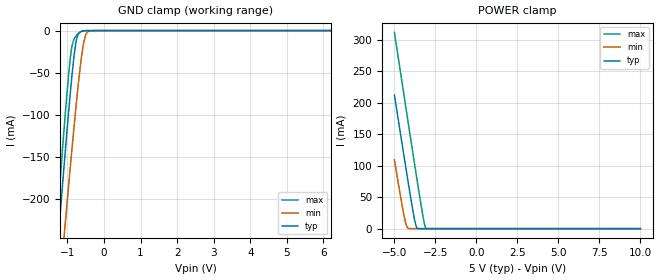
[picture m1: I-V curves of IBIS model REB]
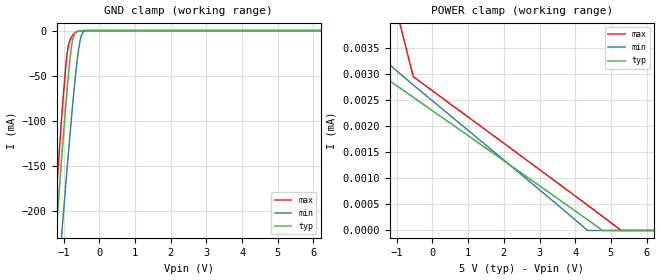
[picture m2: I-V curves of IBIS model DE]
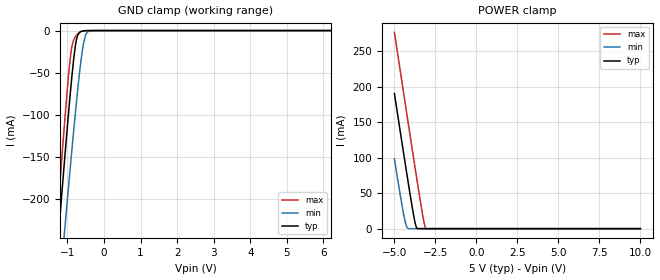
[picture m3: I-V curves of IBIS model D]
|Texas Instruments Incorporated
| THVD1550 5-V RS-485 Transceivers With +/-16-kV IEC ESD Protection
| Marketing part#   Digital Voltage Range   Package-type   #pins
| THVD1550D   4.5V-5.5V   SOIC   8
| THVD1550DGK   4.5V-5.5V   VSSOP   8
[IBIS Ver]   4.1
[File name]   thvd1550.ibs
[Date]   05/26/2017
[File Rev]   1.0
[Source]
| Texas Instruments Incorporated.
| Analog-eLab Design Center, HPA
| 12500 TI Blvd
| Dallas, TX -75243
[Notes]
| Rev 1.0: 05/26/2017
| - Initial version of the model
| - Model generated from simulations in SPECTRE
| - Model matched to SPICE simulation
| - C_comp although listed in numerical order of value are
|   obtained from varying PVT conditions. For PVT conditions for
|   each specific value refer the buffer description under
|   respective [Model]. IBIS model user is responsible for using
|   appropriate C_comp to simulate for Signal Integrity.
[Disclaimer]
| This model is designed as an aid for customers of Texas Instruments.
| TI and its licensors and suppliers make no warranties, either expressed
| or implied, with respect to this  model, including the warranties of
| merchantability or fitness for a particular purpose. The model is
| provided solely on an "as is" basis. The entire risk as to its quality
| and performance is with the customer.
[Copyright]
(C) Copyright 2017 Texas Instruments Incorporated.All rights reserved.
|   THVD1550D
[Component]   THVD1550D
[Manufacturer]  TI
[Package]   |8 SOIC - D package
|   typ   min   max
R_pkg   0   0   0
L_pkg   0   0   0
C_pkg   0   0   0
[Pin]  signal_name model_name   R_pin   L_pin   C_pin
1   R   R   NA   NA   NA
2   _RE   REB   NA   NA   NA
3   DE   DE   NA   NA   NA
4   D   D   NA   NA   NA
5   GND   gnd   NA   NA   NA
6   A   diff   NA   NA   NA
7   B   diff   NA   NA   NA
8   VCC   power   NA   NA   NA
[Diff Pin]  inv_pin  vdiff  tdelay_typ tdelay_min tdelay_max
6   7   0.2   NA   NA   NA
|   THVD1550DGK
[Component]   THVD1550DGK
[Manufacturer]  TI
[Package]   |8 VSSOP - DGK package
|   typ   min   max
R_pkg   0   0   0
L_pkg   0   0   0
C_pkg   0   0   0
[Pin]  signal_name model_name   R_pin   L_pin   C_pin
1   R   R   NA   NA   NA
2   _RE   REB   NA   NA   NA
3   DE   DE   NA   NA   NA
4   D   D   NA   NA   NA
5   GND   gnd   NA   NA   NA
6   A   diff   NA   NA   NA
7   B   diff   NA   NA   NA
8   VCC   power   NA   NA   NA
[Diff Pin]  inv_pin  vdiff  tdelay_typ tdelay_min tdelay_max
6   7   0.2   NA   NA   NA
| Models and submodels in the file (5): REB (Input), DE (Input), D (Input), R (3-state), diff (I/O)
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|   REB Model
[Model]   REB
Model_type   Input
Vinl = 0.5
Vinh = 4.5
|   typ   min   max
C_comp   6.491E-12   5.789E-12   6.939E-12
[Model spec]
|subparameter
Vinl   0.5   0.45   0.55
Vinh   4.5   4.05   4.95
| Where Nom  PVT is Nominal Process, 5V, 27C
|   Fast PVT is Strong Process,  5.5V, -40C
|   Slow PVT is Weak Process,   4.5, 150C
[Voltage Range]   5   4.5   5.5
|Junction Temperature
[Temperature Range]   27   150   -40
[Power Clamp Reference]   5   4.5   5.5
[GND Clamp Reference]   0   0   0
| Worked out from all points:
|   GND clamp passes 1 mA (typ) near -0.62 V on its own axis
|   POWER clamp passes 1 mA (typ) near -3.62 V on its own axis
[GND Clamp]
|   Voltage   I(typ)   I(min)   I(max)
-5V       -2.374A    -2.283A    -2.497A
-1.445V   -351.6mA   -421.6mA   -320.8mA
-1.25V    -244.6mA   -322.9mA   -205.9mA
-1.235V   -236.5mA   -315.3mA   -197.2mA
-1.13V    -180.1mA   -262.9mA   -137.2mA
-1.055V   -140.6mA   -225.9mA   -95.96mA
-905mV    -66.08mA   -153.6mA   -26.41mA
-770mV    -14.61mA   -91.73mA   -6.602mA
-620mV    -1.012mA   -32.37mA   -1.047mA
-485mV    -90.93uA   -3.793mA   -69.28uA
-245mV    -2.701uA   -14.54uA   -2.873uA
10V       0A         0A         0A
[POWER Clamp]
|   Voltage   I(typ)   I(min)   I(max)
-5V       212.6mA    109.6mA    312.1mA
-4.535V   135mA      37.57mA    232.5mA
-4.4V     112.7mA    19.02mA    209.4mA
-4.295V   95.5mA     7.406mA    191.5mA
-4.145V   71.14mA    530.5uA    166mA
-3.86V    26.73mA    342.2nA    117.8mA
-3.71V    7.131mA    36.81nA    92.61mA
-3.59V    443.9uA    20.17nA    72.65mA
-3.245V   0A         0A         17.76mA
-3.155V   0A         0A         6.049mA
-3.065V   0A         0A         462.9uA
10V       0A         0A         0A
|   DE Model
[Model]   DE
Model_type   Input
Vinl = 0.5
Vinh = 4.5
|   typ   min   max
C_comp   4.694E-12   4.505E-12   4.916E-12
[Model spec]
|subparameter
Vinl   0.5   0.45   0.55
Vinh   4.5   4.05   4.95
| Where Nom  PVT is Nominal Process, 5V, 27C
|   Fast PVT is Strong Process,  5.5V, -40C
|   Slow PVT is Weak Process,   4.5, 150C
[Voltage Range]   5   4.5   5.5
|Junction Temperature
[Temperature Range]   27   150   -40
[Power Clamp Reference]   5   4.5   5.5
[GND Clamp Reference]   0   0   0
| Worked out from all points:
|   GND clamp passes 1 mA (typ) near -0.62 V on its own axis
[GND Clamp]
|   Voltage   I(typ)   I(min)   I(max)
-3.6V     -1.572A    -1.544A    -1.635A
-1.319V   -281.9mA   -357.3mA   -245.9mA
-1.209V   -222.2mA   -302.1mA   -182mA
-1.05V    -138.1mA   -223.5mA   -93.32mA
-903.8mV  -65.44mA   -152.9mA   -25.92mA
-855mV    -43.85mA   -130mA     -14.31mA
-769.6mV  -14.41mA   -91.45mA   -6.57mA
-696.4mV  -3.663mA   -60.55mA   -3.123mA
-635.4mV  -1.292mA   -37.49mA   -1.345mA
-513.4mV  -153.7uA   -6.74mA    -127.1uA
-354.8mV  -5.531uA   -160.9uA   -2.275uA
8.6V      0A         0A         0A
[POWER Clamp]
|   Voltage   I(typ)   I(min)   I(max)
-3.6V     287.8uA    4.691uA    64.82mA
-3.222V   3.835uA    4.363uA    11.88mA
-2.99V    3.725uA    4.219uA    9.58uA
-537.8mV  2.553uA    2.79uA     2.948uA
2.707V    998.1nA    947.1nA    1.315uA
4.342V    207.3nA    867.5pA    486.3nA
4.757V    3.159nA    0A         274.4nA
5.306V    0A         0A         0A
8.6V      0A         0A         0A
|   D Model
[Model]   D
Model_type   Input
Vinl = 0.5
Vinh = 4.5
|   typ   min   max
C_comp   4.697E-12   4.504E-12   4.921E-12
[Model spec]
|subparameter
Vinl   0.5   0.45   0.55
Vinh   4.5   4.05   4.95
| Where Nom  PVT is Nominal Process, 5V, 27C
|   Fast PVT is Strong Process,  5.5V, -40C
|   Slow PVT is Weak Process,   4.5, 150C
[Voltage Range]   5   4.5   5.5
|Junction Temperature
[Temperature Range]   27   150   -40
[Power Clamp Reference]   5   4.5   5.5
[GND Clamp Reference]   0   0   0
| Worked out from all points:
|   GND clamp passes 1 mA (typ) near -0.62 V on its own axis
|   POWER clamp passes 1 mA (typ) near -3.64 V on its own axis
[GND Clamp]
|   Voltage   I(typ)   I(min)   I(max)
-5V       -2.374A    -2.283A    -2.496A
-1.445V   -351.5mA   -421.4mA   -320.7mA
-1.25V    -244.5mA   -322.7mA   -205.9mA
-1.235V   -236.4mA   -315.2mA   -197.1mA
-1.13V    -180mA     -262.8mA   -137.2mA
-1.055V   -140.6mA   -225.8mA   -95.89mA
-905mV    -65.99mA   -153.4mA   -26.31mA
-770mV    -14.51mA   -91.62mA   -6.594mA
-620mV    -1.005mA   -32.26mA   -1.047mA
-485mV    -90.93uA   -3.716mA   -69.33uA
-245mV    -2.758uA   -14.06uA   -2.92uA
10V       0A         0A         0A
[POWER Clamp]
|   Voltage   I(typ)   I(min)   I(max)
-5V       190.3mA    98.21mA    276.6mA
-4.505V   116mA      28.78mA    201.2mA
-4.355V   93.68mA    11.05mA    178.4mA
-4.25V    78.2mA     2.751mA    162.5mA
-4.16V    65.06mA    380.8uA    148.9mA
-3.86V    22.95mA    211.4nA    103.7mA
-3.725V   6.92mA     53.48nA    83.57mA
-3.665V   2.229mA    44.46nA    74.66mA
-3.23V    0A         7.317nA    12.98mA
-3.14V    0A         1.289nA    3.33mA
-3.08V    0A         0A         446.2uA
10V       0A         0A         0A
